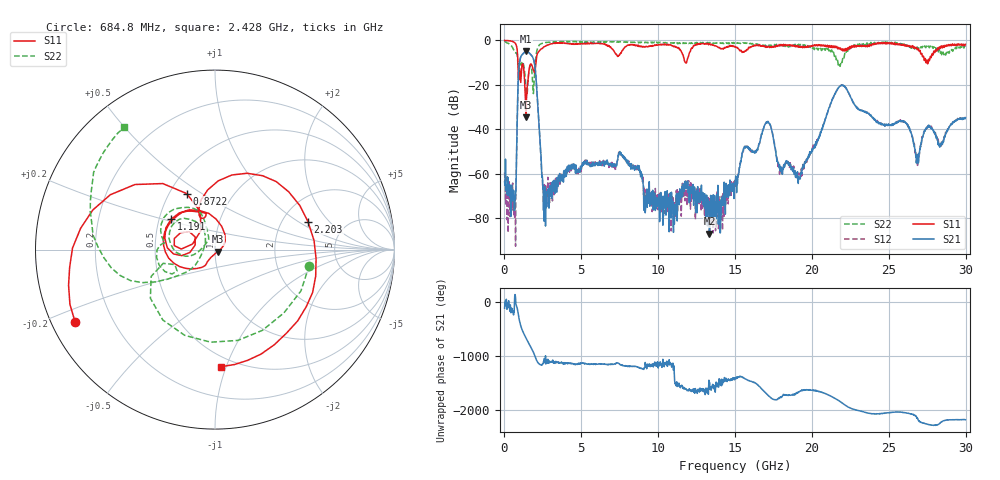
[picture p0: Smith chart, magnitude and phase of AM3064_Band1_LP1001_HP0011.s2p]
# Hz S DB R 50.0
!freq dBS11 angS11 dBS21 angS21 dBS12 angS12 dBS22 angS22
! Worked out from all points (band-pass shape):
!   1600 points, 10 MHz to 29.98 GHz, reference 50 ohm
!   highest |S21| = -4.95 dB at 1.416 GHz (marker M1); lowest = -86.9 dB at 13.34 GHz (marker M2)
!   |S21| within 3 dB of the highest: 1.037 GHz to 1.866 GHz (829 MHz wide, 57.1 % of centre)
!   lowest |S11| = -34.6 dB at 1.397 GHz (marker M3), VSWR 1.04, Z = 51.5 - j1.19 ohm
!   |S11| at or under -10 dB: 876.6 MHz to 2.046 GHz (1.169 GHz wide, 80 % of centre); 11.8025 GHz to 11.84176 GHz (39.26 MHz wide, 0.332 % of centre); 27.50994 GHz to 27.55239 GHz (42.46 MHz wide, 0.154 % of centre)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
!   |S22| runs from -24.3 to -0.4 dB; largest |S21 - S12| = 0.007
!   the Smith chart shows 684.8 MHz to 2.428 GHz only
!   S11 on the Smith chart (normalised r, x): 684.8 MHz: 0.07, -0.24; 872.2 MHz: 0.61, +0.43; 1.191 GHz: 0.58, +0.21; 2.203 GHz: 2.76, +1.21; 2.428 GHz: 0.42, -0.96
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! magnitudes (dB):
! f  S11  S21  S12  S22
! 10 MHz  0.0  -63.5  -59.3  -0.4
! 684.8 MHz  -1.1  -70.8  -71.0  -5.5
! 872.2 MHz  -9.1  -22.8  -22.7  -10.5
! 1.191 GHz  -10.5  -6.2  -6.1  -9.6
! 1.397 GHz  -34.6  -5.0  -5.0  -21.3
! 1.416 GHz  -31.3  -4.9  -4.9  -22.6
! 1.903 GHz  -13.7  -8.7  -8.7  -21.4
! 2.203 GHz  -5.3  -32.8  -32.7  -2.8
! 2.428 GHz  -3.7  -60.7  -58.8  -1.4
! 2.69 GHz  -2.4  -69.9  -66.5  -1.0
! 5.015 GHz  -1.5  -56.7  -57.7  -0.7
! 7.582 GHz  -5.8  -50.5  -51.2  -0.6
! 10 GHz  -2.0  -72.8  -72.3  -0.9
! 13.34 GHz  -1.6  -86.9  -87.6  -1.1
! 15 GHz  -3.0  -64.6  -62.9  -1.5
! 17.07 GHz  -2.9  -37.2  -36.6  -2.4
! 17.99 GHz  -2.4  -58.9  -59.0  -2.2
! 19.99 GHz  -2.7  -49.6  -49.3  -3.1
! 21.9 GHz  -4.3  -20.2  -20.1  -9.4
! 25 GHz  -1.1  -38.2  -37.9  -1.0
! 26.85 GHz  -4.2  -54.5  -54.2  -3.0
! 29.98 GHz  -1.8  -34.9  -35.0  -3.1
